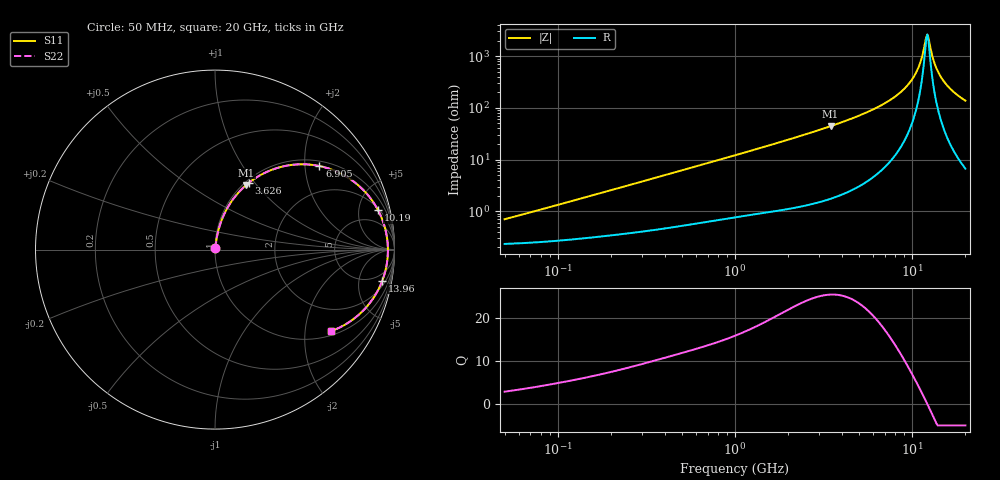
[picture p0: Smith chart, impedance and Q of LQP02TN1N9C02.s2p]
!Murata Part Number: LQP02TN1N9C02
!These Parameters are Measured in Series Mode Connection
!  o--[Z]--o
!Port1  Port2
!  o-------o
!Freq. Start=50[MHz] Stop=20[GHz], 401[Steps]
# Hz S RI R 50
!Freq.(Hz) S11(Real) S11(Imag) S21(Real) S21(Imag) S12(Real) S12(Imag) S22(Real) S22(Imag)
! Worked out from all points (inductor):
!   401 points, 50 MHz to 20 GHz, reference 50 ohm
!   read as one part in series: L = 2.1 nH near 53.89 MHz
!   highest Q = 25.4 at 3.467 GHz (marker M1), where L = 2.03 nH
!   self-resonance near 12.02 GHz
!   S11 on the Smith chart (normalised r, x): 50 MHz: 1.00, +0.01; 3.626 GHz: 1.04, +0.93; 6.905 GHz: 1.14, +2.38; 10.19 GHz: 2.24, +7.76; 13.96 GHz: 3, -10; 20 GHz: 1.13, -2.76
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5e7  0.00238 0.0066  0.9976 -0.0066  0.9976 -0.0066  0.00238 0.0066
1.364002e8  0.00328 0.0175  0.9967 -0.0175  0.9967 -0.0175  0.00328 0.0175
3.721004e8  0.00657 0.0458  0.9934 -0.0458  0.9934 -0.0458  0.00657 0.0458
1e9  0.0217 0.1174  0.9783 -0.1174  0.9783 -0.1174  0.0217 0.1174
2.728004e9  0.1122 0.2958  0.8878 -0.2958  0.8878 -0.2958  0.1122 0.2958
3.466789e9  0.1736 0.3596  0.8264 -0.3596  0.8264 -0.3596  0.1736 0.3596
3.626126e9  0.1886 0.3719  0.8114 -0.3719  0.8114 -0.3719  0.1886 0.3719
5.041459e9  0.3434 0.4538  0.6566 -0.4538  0.6566 -0.4538  0.3434 0.4538
6.905011e9  0.5817 0.4656  0.4183 -0.4656  0.4183 -0.4656  0.5817 0.4656
7.442007e9  0.6494 0.4463  0.3506 -0.4463  0.3506 -0.4463  0.6494 0.4463
8.907419e9  0.8111 0.3471  0.1889 -0.3471  0.1889 -0.3471  0.8111 0.3471
1.019291e10  0.9085 0.2194  0.0915 -0.2194  0.0915 -0.2194  0.9085 0.2194
1.098561e10  0.944 0.1319  0.056 -0.1319  0.056 -0.1319  0.944 0.1319
1.131968e10  0.9533 0.0946  0.0467 -0.0946  0.0467 -0.0946  0.9533 0.0946
1.183995e10  0.9617 0.037  0.0383 -0.037  0.0383 -0.037  0.9617 0.037
1.220001e10  0.9634 -0.0019  0.0366 0.0019  0.0366 0.0019  0.9634 -0.0019
1.238412e10  0.963 -0.0214  0.037 0.0214  0.037 0.0214  0.963 -0.0214
1.314879e10  0.9538 -0.0985  0.0462 0.0985  0.0462 0.0985  0.9538 -0.0985
1.396067e10  0.9326 -0.1723  0.0674 0.1723  0.0674 0.1723  0.9326 -0.1723
1.482269e10  0.9006 -0.2405  0.0994 0.2405  0.0994 0.2405  0.9006 -0.2405
1.621653e10  0.8365 -0.3282  0.1635 0.3282  0.1635 0.3282  0.8365 -0.3282
2e10  0.6488 -0.4537  0.3512 0.4537  0.3512 0.4537  0.6488 -0.4537
